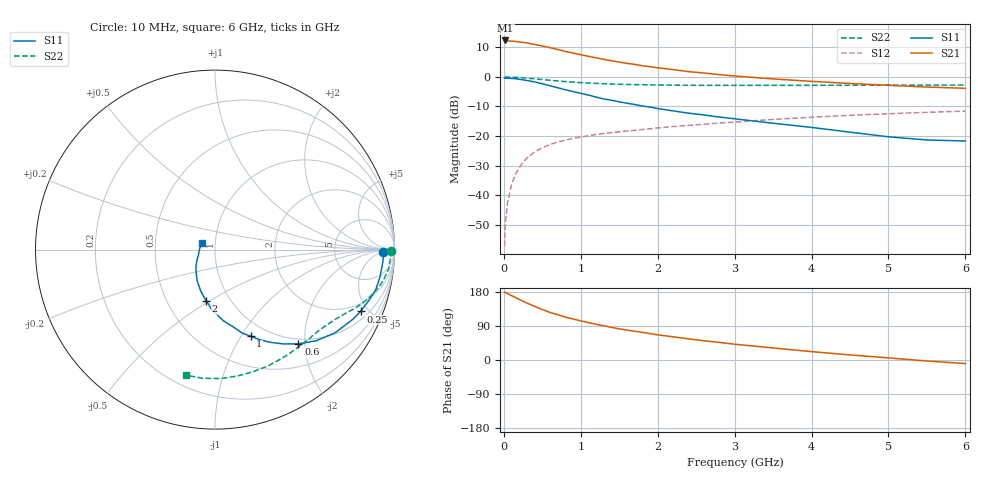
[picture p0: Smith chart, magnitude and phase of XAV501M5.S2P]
! SIEMENS Discrete & RF Semiconductors
! BFY180
! Si NPN RF Bipolar Junction Transistor in MICRO-X
! VCE = 0.5 V  IC = 1.5 mA
! Common Emitter S-Parameters:  May  1997
# GHz  S  MA  R  50
!  f  S11  S21  S12  S22
! GHz  MAG  ANG  MAG  ANG  MAG  ANG  MAG  ANG
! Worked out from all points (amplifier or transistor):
!   36 points, 10 MHz to 6 GHz, reference 50 ohm
!   highest |S21| = 12.2 dB at 20 MHz (marker M1)
!   |S21| within 3 dB of that: start of sweep to 695.1 MHz
!   unconditionally stable (mu >= 1): 1.211 GHz to end of sweep
!   at 250 MHz: K = 0.25, MSG = 20.1 dB, |S12| = -28.8 dB
!   at 1.4 GHz: K = 1.10, MAG = 10.2 dB, |S12| = -18.9 dB
!   at 6 GHz: K = 1.49, MAG = -0.3 dB, |S12| = -11.6 dB
!   S11 on the Smith chart (normalised r, x): 10 MHz: 29, -7; 250 MHz: 1.45, -4.46; 600 MHz: 0.90, -1.87; 1 GHz: 0.83, -1.10; 2 GHz: 0.77, -0.48; 6 GHz: 0.86, +0.06
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0.01  0.9369 -0.9  3.968 179.1  0.0014 81.6  0.9826 -0.3
0.02  0.9402 -2.1  4.055 177.9  0.0035 88.3  0.9829 -0.8
0.05  0.9366 -4.9  3.954 175.1  0.0078 84.4  0.9812 -2.1
0.1  0.932 -9.3  3.964 169.9  0.0152 84.6  0.9755 -4.3
0.15  0.9229 -14.1  3.901 164.9  0.0227 80.2  0.9731 -6.4
0.25  0.8811 -23.0  3.75 155.1  0.0363 74.2  0.9543 -10.3
0.3  0.8595 -27.0  3.695 150.1  0.0425 71.1  0.9413 -12.1
0.4  0.8134 -34.8  3.479 141.5  0.054 66.4  0.9175 -15.3
0.5  0.7574 -42.2  3.276 133.3  0.0634 61.8  0.8912 -18.2
0.6  0.7012 -48.5  3.067 125.5  0.072 58.2  0.8677 -20.6
0.8  0.6007 -59.3  2.652 113.2  0.0853 52.5  0.8231 -24.7
1  0.5214 -67.7  2.337 103.2  0.0963 48.3  0.7902 -28.1
1.1  0.4887 -72.0  2.192 98.6  0.101 46.7  0.7784 -29.6
1.3  0.4199 -79.9  1.947 90.2  0.1103 44.1  0.758 -32.7
1.5  0.3762 -86.3  1.757 82.2  0.1179 41.9  0.7429 -35.6
2  0.2894 -99.9  1.406 66.4  0.1369 38.4  0.724 -43.0
2.2  0.2648 -104.3  1.311 61.2  0.144 36.6  0.7179 -46.0
3  0.1949 -121.0  1.023 41.6  0.1717 30.9  0.7113 -57.6
3.5  0.1641 -130.1  0.914 31.8  0.1902 27.6  0.7123 -65.1
4.5  0.1161 -150.1  0.767 13.4  0.2227 18.8  0.7155 -80.1
5.5  0.0857 176.7  0.667 -2.6  0.2504 9.5  0.7201 -95.5
6  0.0825 153.7  0.635 -9.4  0.262 4.8  0.7184 -103.2
